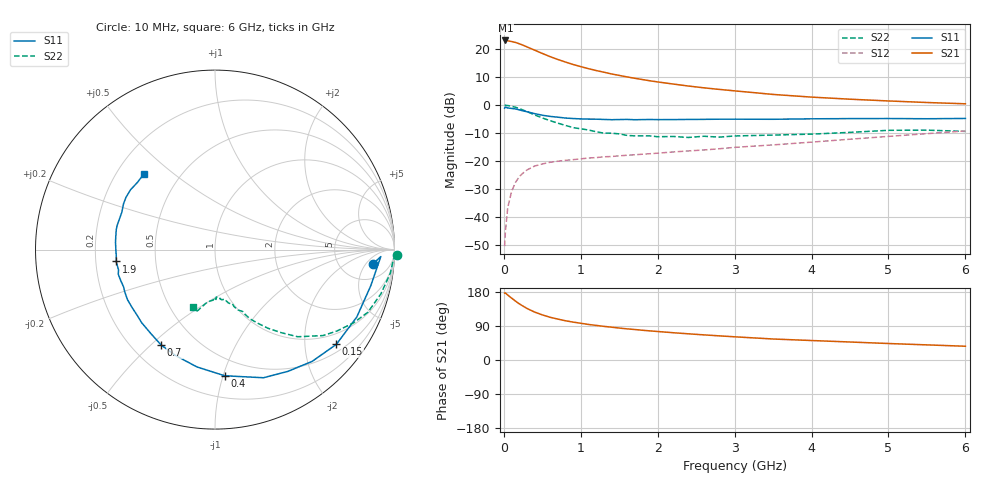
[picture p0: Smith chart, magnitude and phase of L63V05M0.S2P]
!  INFINEON TECHNOLOGIES Small Signal Semiconductors
! BFR380L3 , Si-NPN RF-Transistor in TSLP-3-1
!  Vce=3 V,  Ic=5 mA
! Common Emitter S-Parameters:  07. March 2005
#  GHz  S  MA  R  50
! f  S11  S21  S12  S22
! GHz  Mag  Ang  Mag  Ang  Mag  Ang  Mag  Ang
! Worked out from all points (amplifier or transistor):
!   36 points, 10 MHz to 6 GHz, reference 50 ohm
!   highest |S21| = 23.2 dB at 20 MHz (marker M1)
!   |S21| within 3 dB of that: start of sweep to 360.6 MHz
!   unconditionally stable (mu >= 1): 2.379 GHz to 4.681 GHz
!   at 250 MHz: K = 0.17, MSG = 22.9 dB, |S12| = -24.3 dB
!   at 1.4 GHz: K = 0.76, MSG = 14.8 dB, |S12| = -18.4 dB
!   at 6 GHz: K = 0.93, MSG = 4.9 dB, |S12| = -9.2 dB
!   S11 on the Smith chart (normalised r, x): 10 MHz: 11, -8; 150 MHz: 0.69, -2.75; 400 MHz: 0.36, -1.01; 700 MHz: 0.32, -0.54; 1.9 GHz: 0.29, -0.05; 6 GHz: 0.31, +0.40
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0.01  0.885 -5.1  14.32 176.6  0.003 87.3  1.012 -1.6
0.02  0.9247 -2.4  14.39 176.9  0.0054 88.3  0.9951 -3.2
0.05  0.8909 -13.1  14.18 171.5  0.0145 84.7  0.9857 -7.7
0.1  0.8747 -25.4  13.78 163.5  0.0284 76.6  0.9562 -15.0
0.15  0.8577 -38.0  13.28 155.6  0.0411 70.8  0.9205 -22.3
0.2  0.8251 -49.0  12.57 148.3  0.0525 66.1  0.8728 -27.9
0.25  0.7907 -59.1  11.82 142.1  0.0611 60.6  0.8172 -33.7
0.3  0.7632 -69.3  11.05 136.1  0.0692 57.0  0.7694 -38.5
0.4  0.705 -85.6  9.662 126.5  0.0813 50.9  0.6694 -46.5
0.5  0.6613 -98.8  8.429 119.1  0.0888 47.0  0.5908 -51.5
0.6  0.6296 -110.5  7.399 112.8  0.0951 43.8  0.5289 -56.0
0.7  0.6102 -119.5  6.587 108.0  0.0993 42.8  0.4774 -59.6
0.9  0.5769 -135.1  5.348 100.0  0.106 41.3  0.3975 -65.1
1.1  0.5634 -145.4  4.501 93.8  0.1133 41.4  0.3598 -69.2
1.4  0.55 -158.0  3.62 86.6  0.1207 42.3  0.3151 -73.6
1.9  0.5548 -173.2  2.729 76.8  0.1353 46.1  0.282 -82.6
2.2  0.5522 -179.9  2.39 72.0  0.1454 48.6  0.2756 -84.2
2.8  0.5612 168.6  1.915 63.7  0.166 53.3  0.2682 -91.8
3.5  0.5593 158.2  1.557 55.4  0.1946 56.3  0.2918 -97.0
4.5  0.5751 149.5  1.279 47.5  0.246 60.6  0.3262 -102.8
5.5  0.5717 139.2  1.116 39.9  0.3093 61.0  0.3573 -108.2
6  0.5787 133.2  1.059 36.3  0.3455 60.0  0.3397 -111.0
